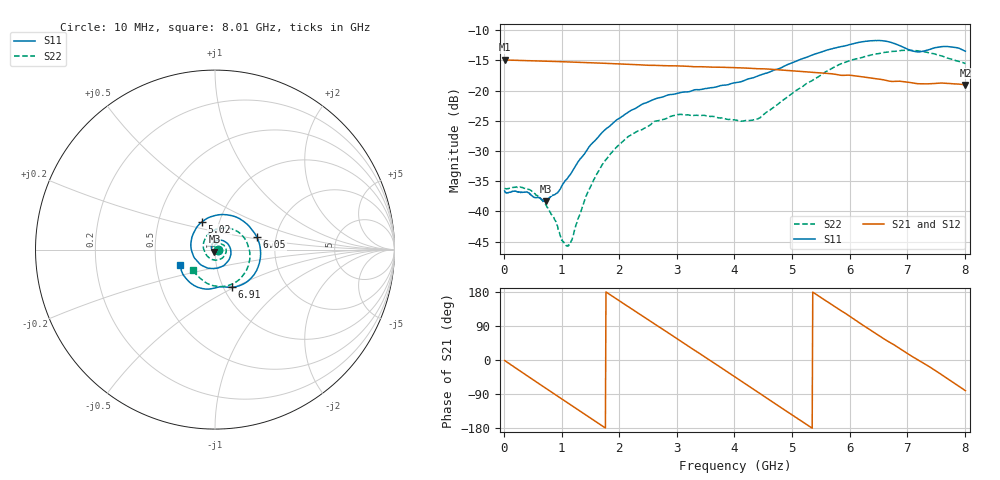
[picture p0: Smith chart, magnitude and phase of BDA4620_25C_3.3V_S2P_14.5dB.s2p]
!Agilent Technologies,E5071B,MY42404982,A.09.10
!Date: Wed May 06 08:51:39 2026
!Data & Calibration Information:
!Freq	S11:SOLT2(ON)	S21:SOLT2(ON)	S12:SOLT2(ON)	S22:SOLT2(ON)
# Hz S RI R 50
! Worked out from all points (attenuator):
!   801 points, 10 MHz to 8.01 GHz, reference 50 ohm
!   highest |S21| = -14.92 dB at 10 MHz (marker M1); lowest = -19.1 dB at 8.01 GHz (marker M2)
!   lowest |S11| = -38.3 dB at 720 MHz (marker M3), VSWR 1.02, Z = 49.7 - j1.16 ohm
!   |S11| at or under -10 dB: start of sweep to end of sweep
!   |S22| runs from -45.7 to -13.3 dB; largest |S21 - S12| = 0.00082
!   S11 on the Smith chart (normalised r, x): 10 MHz: 1.03, -0.00; 5.02 GHz: 0.83, +0.26; 6.05 GHz: 1.59, +0.23; 6.91 GHz: 1.10, -0.49; 8.01 GHz: 0.67, -0.12
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1e7  0.0147 -0.000983  0.1795 -0.00384  0.1797 -0.00392  0.0155 -0.000683
4.3e8  0.00906 -0.0111  0.1261 -0.1238  0.1261 -0.1241  0.0136 -0.00685
7.2e8  -0.00301 -0.0117  0.0478 -0.1684  0.0479 -0.1687  0.00682 -0.00927
1.09e9  -0.0185 0.00127  -0.0641 -0.1603  -0.0643 -0.1605  -0.00417 -0.00308
1.17e9  -0.0198 0.00678  -0.0859 -0.1492  -0.0861 -0.1494  -0.00574 -0.000426
1.35e9  -0.0202 0.0197  -0.1273 -0.114  -0.1274 -0.1141  -0.00775 0.00707
1.59e9  -0.0112 0.0374  -0.1612 -0.0512  -0.1615 -0.0512  -0.0058 0.0187
1.89e9  0.0137 0.0519  -0.163 0.0364  -0.1632 0.0364  0.00567 0.031
2.68e9  0.0869 0.00243  0.00421 0.1611  0.00442 0.1613  0.0532 0.0184
3.4e9  0.0353 -0.0953  0.1507 0.0451  0.151 0.045  0.0458 -0.0422
4.01e9  -0.0823 -0.0817  0.1098 -0.1087  0.1099 -0.1091  -0.0214 -0.053
4.42e9  -0.1327 0.00356  0.0105 -0.1512  0.0102 -0.1513  -0.058 -0.0102
5.02e9  -0.0724 0.1543  -0.122 -0.0798  -0.1223 -0.0798  -0.0331 0.09
5.35e9  0.0269 0.1947  -0.1415 -2.97e-05  -0.1417 -9.5e-05  0.0287 0.1174
5.66e9  0.1339 0.174  -0.1182 0.0711  -0.1182 0.0714  0.097 0.1138
6.05e9  0.2334 0.0691  -0.0458 0.1249  -0.0459 0.1251  0.1722 0.0508
6.37e9  0.2499 -0.0635  0.0262 0.1243  0.0263 0.1244  0.1947 -0.0277
6.68e9  0.1783 -0.1794  0.0803 0.0889  0.0805 0.0893  0.1772 -0.1104
6.91e9  0.0953 -0.2099  0.1065 0.0528  0.1068 0.053  0.1406 -0.1624
7.19e9  0.027 -0.207  0.1139 -0.000154  0.1142 -0.000139  0.0666 -0.2026
7.57e9  -0.082 -0.214  0.0934 -0.0677  0.0936 -0.0677  -0.0371 -0.191
8.01e9  -0.1939 -0.0841  0.0177 -0.1097  0.0179 -0.1099  -0.12 -0.1155
